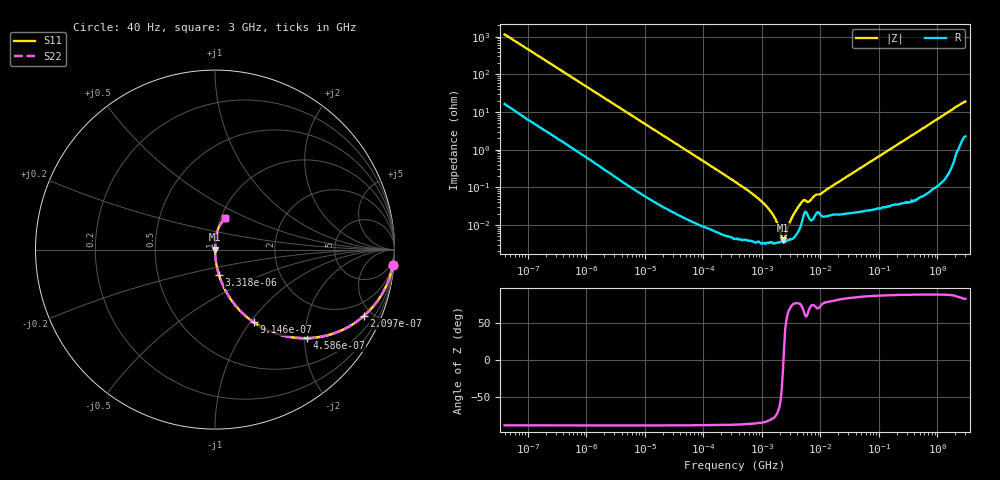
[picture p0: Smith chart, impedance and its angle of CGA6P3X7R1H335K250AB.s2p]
! S-parameter Generated by TDK Corporation
! Copyright(C) 2015 TDK Corporation.
! All Rights Reserved.
! TDK P/N: CGA6P3X7R1H335K250AB (Multilayer Ceramic Chip Capacitors)
! Property: C=3.3uF
! Size(LxWxT): 3.2x2.5x2.5mm, 0.126x0.098x0.098inches
! Model Type: s2p (Touchstone File Format Version 1.0)
! Frequency: DC=Yes Start=0.00004MHz Stop=3000MHz 396points Log-sweep
! Note: This model was converted from impedance.
! Model Generated on Jun. 23, 2015
! Hash(MD5):
! Port Assignments:
!  1 ---| |--- 2
! Applicable Conditions:
!  Temperature = 25 degC
!  DC Bias Voltage = 0 V
!  Small Signal Operation
! Terms and conditions regarding TDK Simulation Models
! (1)This simulation model is being provided solely for informational purposes. Please refer to the specifications of the products in terms of detailed characteristics of such products.
! (2)In no event shall TDK Corporation of any of its subsidiaries be liable for any loss or damage arising, directly or indirectly,
!  From any information contained in this simulation model, including, but not limited to loss or damages arising from any inaccuracies, omissions or errors in connection with such information.
! (3)Any and all copyrights on this simulation model are owned by TDK Corporation.
!  Duplication or redistribution of this simulation model without prior written permission from TDK Corporation is prohibited.
! (4)This simulation model is subject to any modification or change without any prior notice.
! (5)Neither TDK Corporation nor any of its subsidiaries shall make any warranty, express or implied,
!  Including but not limited to the correctness, implied warranties of merchantability and fitness for a particular purpose with respect to this simulation models.
! (6)The use of this simulation model shall be deemed to have consented to the terms and conditions hereof.
# MHz S MA R 50
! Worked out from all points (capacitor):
!   395 points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, 40 Hz to 3 GHz, reference 50 ohm
!   read as one part in series: C = 3.47 uF near 41.88 Hz
!   lowest |Z| = 3.91 mohm at 2.286 MHz (marker M1)
!   series resonance near 2.334 MHz, so ESL is about 1.3 nH
!   S11 on the Smith chart (normalised r, x): 40 Hz: 1, -23; 209.7 Hz: 1.06, -4.46; 458.6 Hz: 1.03, -2.05; 914.6 Hz: 1.01, -1.04; 3.318 kHz: 1.00, -0.29; 3 GHz: 1.05, +0.38
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4e-05  0.995 -5.0  0.08685 84.2  0.08685 84.2  0.995 -5.0
0.0001100992  0.9701 -13.3  0.2299 75.9  0.2299 75.9  0.9701 -13.3
0.000209705  0.9078 -24.0  0.4073 65.2  0.4073 65.2  0.9078 -24.0
0.0004585594  0.7116 -43.9  0.6931 45.4  0.6931 45.4  0.7116 -43.9
0.000834128  0.491 -59.8  0.8648 29.4  0.8648 29.4  0.491 -59.8
0.0009145504  0.4578 -62.0  0.883 27.2  0.883 27.2  0.4578 -62.0
0.001588756  0.2866 -72.6  0.9544 16.7  0.9544 16.7  0.2866 -72.6
0.003317849  0.1434 -81.1  0.9879 8.2  0.9879 8.2  0.1434 -81.1
0.01739424  0.0281 -87.7  0.9993 1.6  0.9993 1.6  0.0281 -87.7
0.3464102  0.001417 -88.2  1 0.1  1 0.1  0.001417 -88.2
0.9105995  0.0004745 -85.7  1 0.0  1 0.0  0.0004745 -85.7
1.442786  0.0002199 -81.1  1 0.0  1 0.0  0.0002199 -81.1
1.901634  9.736e-05 -69.1  1 0.0  1 0.0  9.736e-05 -69.1
2.286002  3.91e-05 -14.2  1 0.0  1 0.0  3.91e-05 -14.2
2.877491  0.0001034 67.6  1 -0.0  1 -0.0  0.0001034 67.6
3.622024  0.0002149 77.0  1 -0.0  1 -0.0  0.0002149 77.0
4.998775  0.0004387 70.0  0.9998 -0.0  0.9998 -0.0  0.0004387 70.0
6.292177  0.0004118 67.1  0.9998 -0.0  0.9998 -0.0  0.0004118 67.1
7.22376  0.0005162 74.8  0.9999 -0.0  0.9999 -0.0  0.0005162 74.8
150.6385  0.009949 87.6  0.9996 -0.6  0.9996 -0.6  0.009949 87.6
906.6656  0.05863 85.7  0.9973 -3.4  0.9973 -3.4  0.05863 85.7
3000  0.1826 72.7  0.9618 -10.4  0.9618 -10.4  0.1826 72.7
